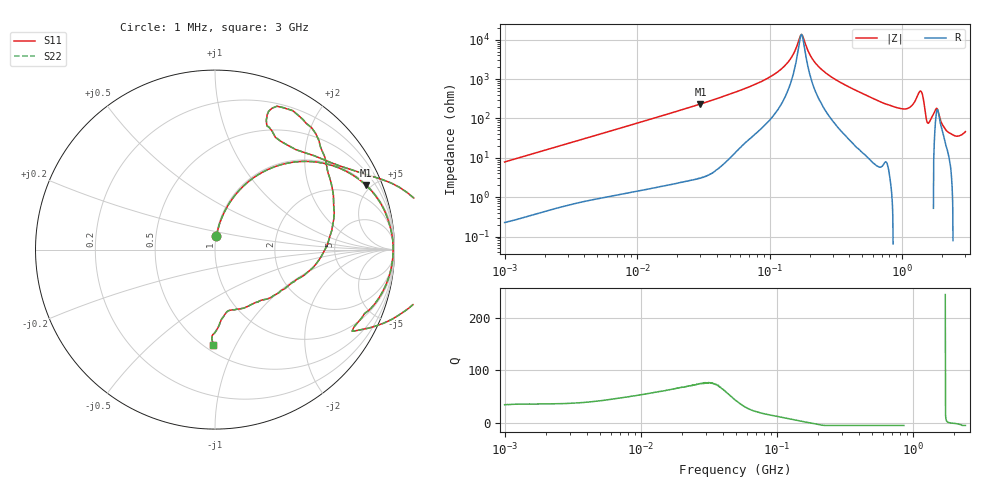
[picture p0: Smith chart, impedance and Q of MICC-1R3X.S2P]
!s-Parameter Generated by FASTRON Sdn. Bhd.
!FASTRON P/N : MICC-1R3X
!Keysight Technologies,E4991B,MY54100416,A.01.15
!Date: Fri Aug 28 09:08:54 2026
!Version  : Rev00 Fri Aug 28 09:08:54 2026
!Data & Calibration Information:
!PortZ  Port1:50+j0  Port2:50+j0
!When reading, reference impedance value at option line is always used.
! Remarks : This data is being provided solely for informational purposes.
!Freq	S11	S21	S12	S22
# Hz S dB R 50
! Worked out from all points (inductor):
!   1601 points, 1 MHz to 3 GHz, reference 50 ohm
!   read as one part in series: L = 1.24 uH near 1.041 MHz
!   highest Q = 76.1 at 30.05 MHz (marker M1), where L = 1.24 uH
!   self-resonance near 173.1 MHz
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1000000  -22.17 83.9  -0.05 -4.5  -0.05 -4.5  -22.17 83.9
3804036  -11.11 72.4  -0.41 -16.2  -0.41 -16.2  -11.11 72.4
1.447069e7  -2.69 41.9  -3.51 -47.2  -3.51 -47.2  -2.69 41.9
3.00453e7  -0.77 23.1  -8.13 -66.2  -8.13 -66.2  -0.77 23.1
5.477226e7  -0.25 12.1  -13.56 -76.2  -13.56 -76.2  -0.25 12.1
1.207609e8  -0.08 3.3  -24.86 -79.6  -24.86 -79.6  -0.08 3.3
1.460522e8  -0.07 1.5  -31.11 -73.6  -31.11 -73.6  -0.07 1.5
1.731398e8  -0.06 0.0  -42.70 -6.1  -42.70 -6.1  -0.06 0.0
2.083556e8  -0.07 -1.6  -30.71 73.7  -30.71 73.7  -0.07 -1.6
3.188066e8  -0.11 -6.0  -19.60 80.0  -19.60 80.0  -0.11 -6.0
7.925923e8  -0.88 -24.1  -7.77 64.7  -7.77 64.7  -0.88 -24.1
1.054198e9  -1.01 -30.7  -5.82 62.7  -5.82 62.7  -1.01 -30.7
1.200675e9  -0.10 -25.6  -7.12 75.7  -7.12 75.7  -0.10 -25.6
1.294266e9  1.17 -15.5  -9.81 108.6  -9.81 108.6  1.17 -15.5
1.374365e9  1.95 0.0  -12.00 -180.0  -12.00 -180.0  1.95 0.0
1.430499e9  1.17 14.6  -10.26 -110.5  -10.26 -110.5  1.17 14.6
1.542004e9  -3.02 58.4  -1.20 -43.7  -1.20 -43.7  -3.02 58.4
1.613037e9  -1.21 66.6  0.28 -50.7  0.28 -50.7  -1.21 66.6
1.818868e9  -3.47 12.0  -8.61 -22.1  -8.61 -22.1  -3.47 12.0
1.970482e9  -6.48 -22.2  -4.60 17.7  -4.60 17.7  -6.48 -22.2
2.543347e9  -9.17 -76.1  -0.21 20.2  -0.21 20.2  -9.17 -76.1
3e9  -5.50 -91.3  1.16 27.7  1.16 27.7  -5.50 -91.3
